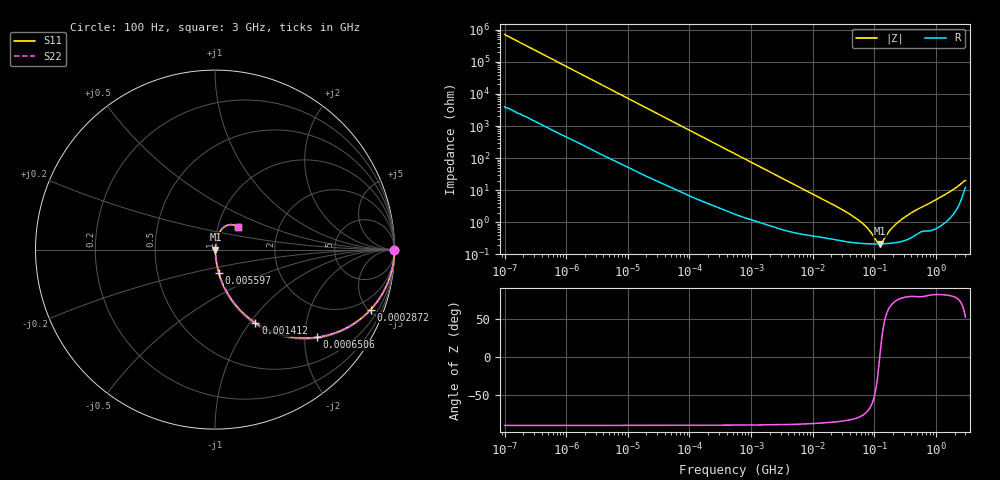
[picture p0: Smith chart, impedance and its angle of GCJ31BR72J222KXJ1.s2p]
!Murata Part Number: GCJ31BR72J222KXJ1
!These Parameters are Measured in Series Mode Connection
!Data Generated on Mar 13, 2026
!  o--ll--o
!Port1  Port2
!  o------o
!Operation Temp=25[degC], DC Bias Voltage=0[V]
!Freq. Start=100[Hz] Stop=3[GHz] 401[Steps]
# Hz S RI R 50
!Freq.(Hz) S11(Real) S11(Imag) S21(Real) S21(Imag) S12(Real) S12(Imag) S22(Real) S22(Imag)
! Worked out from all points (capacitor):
!   401 points, 100 Hz to 3 GHz, reference 50 ohm
!   read as one part in series: C = 2.22 nF near 109 Hz
!   lowest |Z| = 212 mohm at 124.1 MHz (marker M1)
!   series resonance near 122.1 MHz, so ESL is about 770 pH
!   S11 on the Smith chart (normalised r, x): 100 Hz: open; 287.2 kHz: 1.06, -5.17; 650.6 kHz: 1.03, -2.30; 1.412 MHz: 1.02, -1.06; 5.597 MHz: 1.01, -0.27; 3 GHz: 1.24, +0.32
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100  1 -0.00014  8e-07 0.00014  8e-07 0.00014  1 -0.00014
1788  1 -0.00247  2.22e-05 0.00247  2.22e-05 0.00247  1 -0.00247
31977  0.9978 -0.0434  0.00223 0.0434  0.00223 0.0434  0.9978 -0.0434
106717  0.9783 -0.1411  0.0217 0.1411  0.0217 0.1411  0.9783 -0.1411
287190  0.8672 -0.3337  0.1328 0.3337  0.1328 0.3337  0.8672 -0.3337
547723  0.648 -0.4711  0.352 0.4711  0.352 0.4711  0.648 -0.4711
650627  0.5677 -0.4886  0.4323 0.4886  0.4323 0.4886  0.5677 -0.4886
1411895  0.225 -0.4085  0.775 0.4085  0.775 0.4085  0.225 -0.4085
2579298  0.0842 -0.2666  0.9158 0.2666  0.9158 0.2666  0.0842 -0.2666
5597215  0.0223 -0.1321  0.9777 0.1321  0.9777 0.1321  0.0223 -0.1321
9794414  0.0097 -0.0767  0.9903 0.0767  0.9903 0.0767  0.0097 -0.0767
2.872754e7  0.00328 -0.0257  0.9967 0.0257  0.9967 0.0257  0.00328 -0.0257
5.248048e7  0.00238 -0.0123  0.9976 0.0123  0.9976 0.0123  0.00238 -0.0123
7.405258e7  0.00218 -0.00676  0.9978 0.00676  0.9978 0.00676  0.00218 -0.00676
1.090876e8  0.0021 -0.00147  0.9979 0.00147  0.9979 0.00147  0.0021 -0.00147
1.241234e8  0.00211 0.000215  0.9979 -0.000215  0.9979 -0.000215  0.00211 0.000215
1.352818e8  0.00212 0.00134  0.9979 -0.00134  0.9979 -0.00134  0.00212 0.00134
1.751444e8  0.00221 0.0048  0.9978 -0.0048  0.9978 -0.0048  0.00221 0.0048
2.36726e8  0.00244 0.00927  0.9976 -0.00927  0.9976 -0.00927  0.00244 0.00927
3.640608e8  0.0033 0.0172  0.9967 -0.0172  0.9967 -0.0172  0.0033 0.0172
1.789813e9  0.0235 0.0917  0.9765 -0.0917  0.9765 -0.0917  0.0235 0.0917
3e9  0.1259 0.1253  0.8741 -0.1253  0.8741 -0.1253  0.1259 0.1253
